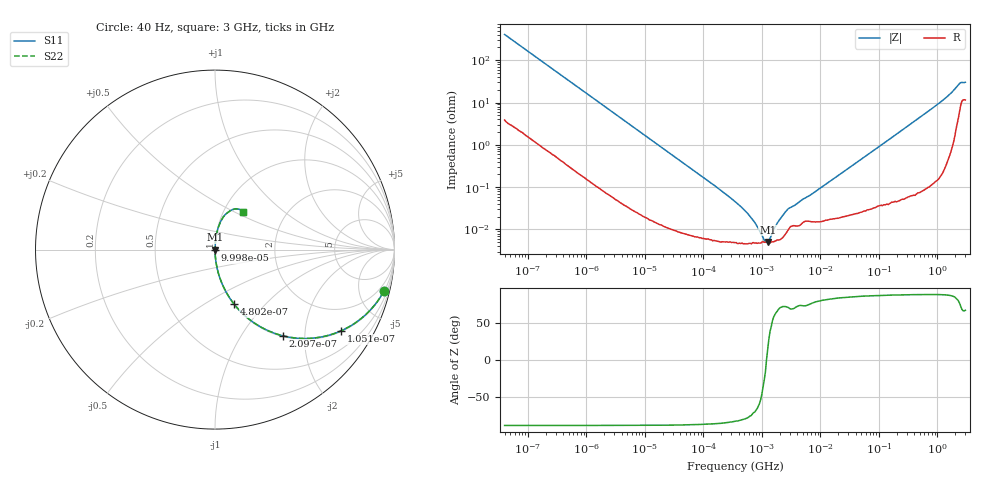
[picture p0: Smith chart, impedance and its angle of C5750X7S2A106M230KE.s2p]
! S-parameter Generated by TDK Corporation
! Copyright(C) 2015 TDK Corporation.
! All Rights Reserved.
! TDK P/N: C5750X7S2A106M230KE (Multilayer Ceramic Chip Capacitors)
! Property: C=10uF
! Size(LxWxT): 5.7x5x2.3mm, 0.224x0.197x0.091inches
! Model Type: s2p (Touchstone File Format Version 1.0)
! Frequency: DC=Yes Start=0.00004MHz Stop=3000MHz 396points Log-sweep
! Note: This model was converted from impedance.
! Model Generated on Jun. 23, 2015
! Hash(MD5):
! Port Assignments:
!  1 ---| |--- 2
! Applicable Conditions:
!  Temperature = 25 degC
!  DC Bias Voltage = 0 V
!  Small Signal Operation
! Terms and conditions regarding TDK Simulation Models
! (1)This simulation model is being provided solely for informational purposes. Please refer to the specifications of the products in terms of detailed characteristics of such products.
! (2)In no event shall TDK Corporation of any of its subsidiaries be liable for any loss or damage arising, directly or indirectly,
!  From any information contained in this simulation model, including, but not limited to loss or damages arising from any inaccuracies, omissions or errors in connection with such information.
! (3)Any and all copyrights on this simulation model are owned by TDK Corporation.
!  Duplication or redistribution of this simulation model without prior written permission from TDK Corporation is prohibited.
! (4)This simulation model is subject to any modification or change without any prior notice.
! (5)Neither TDK Corporation nor any of its subsidiaries shall make any warranty, express or implied,
!  Including but not limited to the correctness, implied warranties of merchantability and fitness for a particular purpose with respect to this simulation models.
! (6)The use of this simulation model shall be deemed to have consented to the terms and conditions hereof.
# MHz S MA R 50
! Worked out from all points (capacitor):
!   395 points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, 40 Hz to 3 GHz, reference 50 ohm
!   read as one part in series: C = 9.8 uF near 41.88 Hz
!   lowest |Z| = 5.03 mohm at 1.257 MHz (marker M1)
!   series resonance near 1.197 MHz, so ESL is about 1.8 nH
!   S11 on the Smith chart (normalised r, x): 40 Hz: 1.08, -8.11; 105.1 Hz: 1.03, -3.09; 209.7 Hz: 1.01, -1.56; 480.2 Hz: 1.01, -0.68; 99.98 kHz: 1.00, -0.00; 3 GHz: 1.23, +0.56
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4e-05  0.9688 -13.8  0.2389 75.6  0.2389 75.6  0.9688 -13.8
6.63624e-05  0.9227 -22.1  0.3769 67.3  0.3769 67.3  0.9227 -22.1
0.000105147  0.8363 -32.7  0.5405 56.7  0.5405 56.7  0.8363 -32.7
0.000209705  0.6117 -51.7  0.7853 37.7  0.7853 37.7  0.6117 -51.7
0.0003173189  0.4568 -62.3  0.8852 27.2  0.8852 27.2  0.4568 -62.3
0.0004801568  0.3227 -70.6  0.9435 18.8  0.9435 18.8  0.3227 -70.6
0.000834128  0.1936 -78.3  0.9793 11.2  0.9793 11.2  0.1936 -78.3
0.002759985  0.06016 -86.0  0.9976 3.4  0.9976 3.4  0.06016 -86.0
0.01739424  0.009673 -88.7  0.9998 0.6  0.9998 0.6  0.009673 -88.7
0.09998367  0.001693 -87.8  0.9999 0.1  0.9999 0.1  0.001693 -87.8
0.3464102  0.0004547 -83.8  1 0.0  1 0.0  0.0004547 -83.8
0.5747153  0.0002359 -78.8  1 0.0  1 0.0  0.0002359 -78.8
0.8696408  0.0001048 -62.9  1 0.0  1 0.0  0.0001048 -62.9
1.256723  5.033e-05 15.3  1 -0.0  1 -0.0  5.033e-05 15.3
1.581893  9.712e-05 58.3  0.9999 -0.0  0.9999 -0.0  9.712e-05 58.3
2.748062  0.0002988 71.8  0.9999 -0.0  0.9999 -0.0  0.0002988 71.8
7.22376  0.0006949 77.4  0.9998 -0.0  0.9998 -0.0  0.0006949 77.4
150.6385  0.01353 87.5  0.9995 -0.8  0.9995 -0.8  0.01353 87.5
572.2325  0.0509 86.1  0.9979 -2.9  0.9979 -2.9  0.0509 86.1
1436.554  0.1331 80.8  0.9876 -7.6  0.9876 -7.6  0.1331 80.8
2383.329  0.2558 62.9  0.9122 -14.5  0.9122 -14.5  0.2558 62.9
3000  0.2619 53.6  0.8705 -14.0  0.8705 -14.0  0.2619 53.6
